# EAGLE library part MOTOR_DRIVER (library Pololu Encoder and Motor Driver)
DRV8835 Dual Motor Driver Carrier
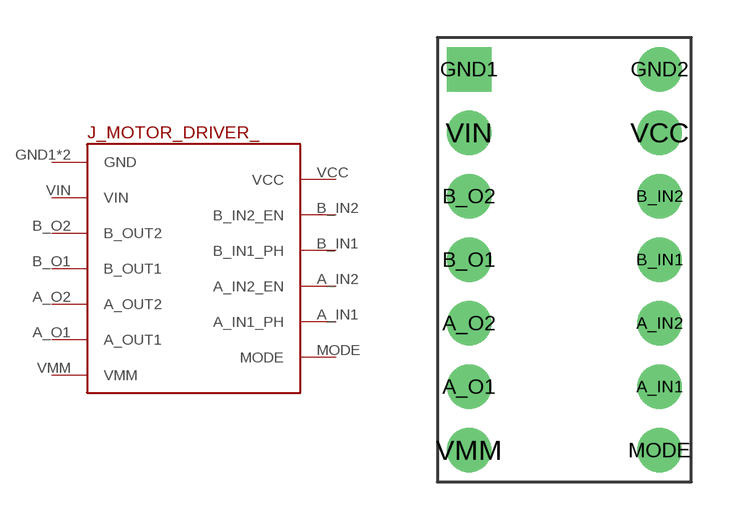
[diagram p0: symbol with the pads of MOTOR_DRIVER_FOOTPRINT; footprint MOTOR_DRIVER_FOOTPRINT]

Designator prefix J_MOTOR_DRIVER_

## MOTOR_DRIVER  [MOTOR_DRIVER_FOOTPRINT]
A_IN1  A_IN1_PH
A_IN2  A_IN2_EN
A_O1  A_OUT1
A_O2  A_OUT2
B_IN1  B_IN1_PH
B_IN2  B_IN2_EN
B_O1  B_OUT1
B_O2  B_OUT2
GND1  GND
GND2  GND
MODE  MODE
VCC  VCC
VIN  VIN
VMM  VMM

## Footprint MOTOR_DRIVER_FOOTPRINT (pad centres in mm)
DRV8835 Dual Motor Driver Carrier Footprint
drill 0.9 pad 1.778: A_IN1 3.81,-5.08; A_IN2 3.81,-2.54; A_O1 -3.81,-5.08; A_O2 -3.81,-2.54; B_IN1 3.81,0; B_IN2 3.81,2.54; B_O1 -3.81,0; B_O2 -3.81,2.54; GND2 3.81,7.62; MODE 3.81,-7.62; VCC 3.81,5.08; VIN -3.81,5.08; VMM -3.81,-7.62
drill 0.9 pad 1.778 square: GND1 -3.81,7.62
